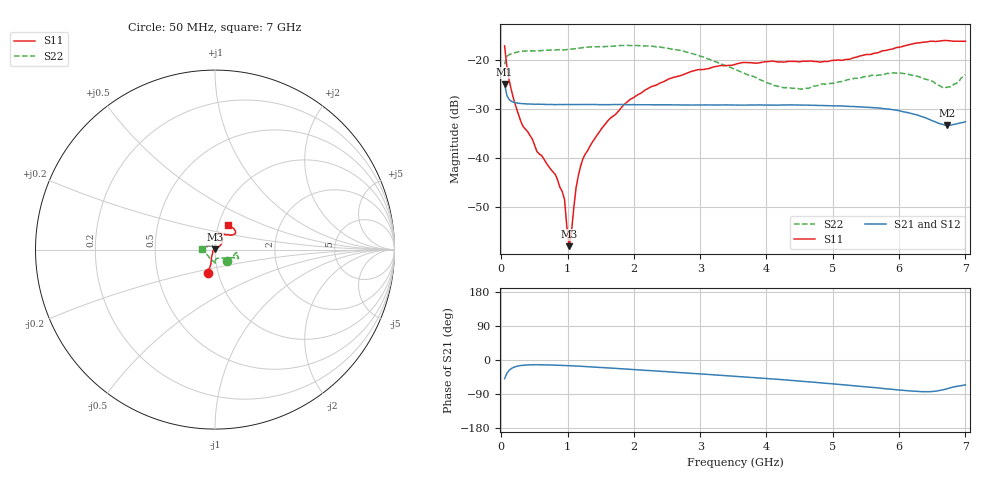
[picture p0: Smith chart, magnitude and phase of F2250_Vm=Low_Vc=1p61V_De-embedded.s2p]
! Integrated Device Technology
! Corporate Headquarters
! 6024 Silver Creek Valley Road
! San Jose, CA 95138  USA
! Phone:  1-408-284-8200
! Toll Free:  1-800-223-1366
! Webpage:  http://www.idt.com/
! Timing and RF Division
! 515 Groton Road, Suite 102
! Westford, MA 01886-6024
! Device:  F2250
! Description: Voltage Variable RF Attenuator
! Frequency:  50.0 -  6000.00 MHz
! Package:  3x3 mm Thin QFN Plastic Package: 16 pin
! Ports:  2 RF, 3 DC
!  Pin  1  = GND
!  Pin  2  = NC
!  Pin  3  = RF1  = Port 1
!  Pin  4  = NC
!  Pin  5  = GND
!  Pin  6  = GND
!  Pin  7  = GND
!  Pin  8  = GND
!  Pin  9  = NC
!  Pin 10  = RF2  = Port 2
!  Pin 11  = NC
!  Pin 12  = GND
!  Pin 13  = GND
!  Pin 14  = VCNTRL
!  Pin 15  = VDD
!  Pin 16  = VMODE
! Vcntrl:  1.610 Volts
! Vmode:  +0.000 Volts
! Vdd:  +3.30  Volts
! Current:  1.189 mA
! Data:  The device was measured on a the F2250 evaluation board which has
!  individual transmission lines to the RF pins.  Data was collected
!  using a calibrated network analyzer.  The evaluation board was
!  de-embedded using a TRL calibration technique.
!  The reference plane is the edge of the package pin.
! Misc:  SN 10
!  Action Tracker AT0258
! Date Measured:  2014-11-26
! Date:  2015-10-15  MJV
! Note:
!  Integrated Device Technology supplies this data as a sample of measured
!  data at the package pin for this product.  Your particular data for this
!  product may vary.
!  Data was taken at 25 degrees C.
!  Integrated Device Technology reserves the right to change this data at anytime.
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# GHz S dB R 50
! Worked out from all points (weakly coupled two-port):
!   201 points, 50 MHz to 7 GHz, reference 50 ohm
!   highest |S21| = -25.00 dB at 50 MHz (marker M1); lowest = -33.3 dB at 6.722 GHz (marker M2)
!   lowest |S11| = -58.1 dB at 1.023 GHz (marker M3), VSWR 1.00, Z = 49.9 + j0.112 ohm
!   |S11| at or under -10 dB: start of sweep to end of sweep
!   |S22| runs from -26.0 to -17.1 dB; largest |S21 - S12| = 0.00019
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0.05  -17.16 -107.4  -25.00 -49.3  -24.99 -49.3  -20.91 -43.7
0.1195  -24.24 -109.7  -28.13 -27.0  -28.13 -27.0  -18.94 -12.7
0.29325  -32.53 -123.1  -28.92 -14.6  -28.95 -14.6  -18.25 -8.5
0.5365  -38.70 -149.1  -29.06 -12.5  -29.05 -12.5  -18.17 -8.9
0.8145  -43.40 175.2  -29.16 -13.6  -29.13 -13.6  -18.00 -12.6
0.91875  -46.88 156.3  -29.15 -14.3  -29.15 -14.3  -17.93 -14.2
0.9535  -48.48 174.9  -29.13 -14.5  -29.14 -14.5  -18.00 -14.4
1.023  -58.06 116.7  -29.12 -15.0  -29.17 -15.0  -17.85 -14.6
1.05775  -55.22 77.0  -29.14 -15.3  -29.18 -15.3  -17.82 -14.8
1.12725  -46.18 40.8  -29.14 -15.9  -29.15 -15.9  -17.69 -15.8
1.2315  -40.19 32.9  -29.12 -16.9  -29.13 -16.9  -17.50 -17.3
1.6485  -31.87 37.5  -29.16 -21.3  -29.13 -21.3  -17.26 -19.2
1.9265  -28.28 38.5  -29.16 -24.4  -29.15 -24.4  -17.07 -20.2
2.37825  -24.87 45.3  -29.20 -29.5  -29.20 -29.5  -17.37 -21.3
2.93425  -22.11 58.6  -29.22 -35.9  -29.22 -35.9  -18.94 -23.7
3.525  -20.94 71.6  -29.26 -42.9  -29.26 -43.0  -21.97 -36.3
4.22  -20.43 77.8  -29.23 -51.6  -29.23 -51.6  -25.59 -62.8
4.7065  -20.33 71.8  -29.29 -58.6  -29.27 -58.6  -25.39 -82.6
5.85325  -17.90 39.9  -30.08 -76.8  -30.09 -76.8  -22.79 -88.4
6.2355  -16.65 38.9  -31.14 -82.6  -31.13 -82.6  -23.23 -95.1
6.722  -16.07 49.7  -33.35 -75.8  -33.35 -75.8  -25.57 -145.7
7  -16.22 62.9  -32.63 -65.6  -32.60 -65.8  -23.02 178.0
